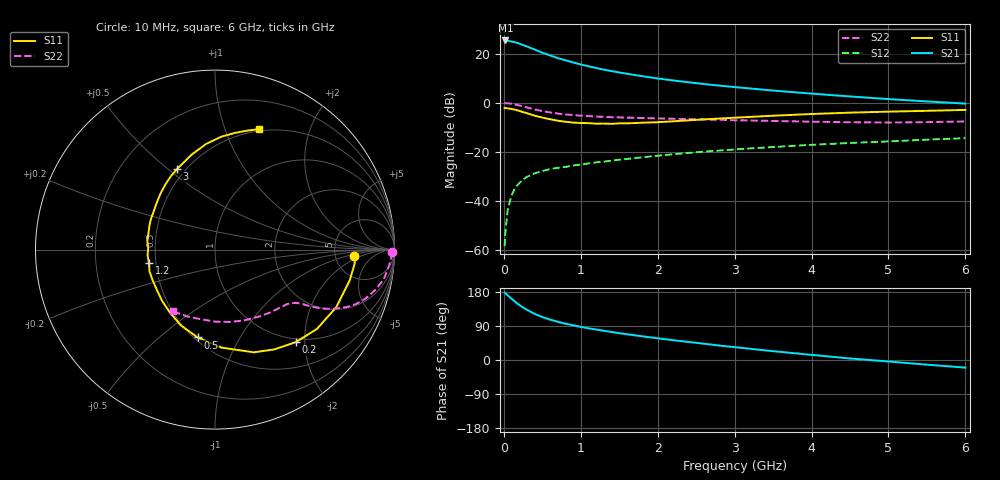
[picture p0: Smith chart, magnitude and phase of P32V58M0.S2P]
! SIEMENS Small Signal Semiconductors
! BFP181
! Si NPN RF Bipolar Junction Transistor in SOT143
! VCE = 2.5 V  IC = 8 mA
! Common Emitter S-Parameters:  March  1996
# GHz  S  MA  R  50
!  f  S11  S21  S12  S22
! GHz  MAG  ANG  MAG  ANG  MAG  ANG  MAG  ANG
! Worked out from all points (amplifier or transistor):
!   36 points, 10 MHz to 6 GHz, reference 50 ohm
!   highest |S21| = 25.4 dB at 20 MHz (marker M1)
!   |S21| within 3 dB of that: start of sweep to 344 MHz
!   unconditionally stable (mu >= 1): 1.239 GHz to end of sweep
!   at 250 MHz: K = 0.30, MSG = 27.4 dB, |S12| = -31.2 dB
!   at 1.4 GHz: K = 1.06, MAG = 16.8 dB, |S12| = -23.6 dB
!   at 6 GHz: K = 1.02, MAG = 6.3 dB, |S12| = -14.4 dB
!   S11 on the Smith chart (normalised r, x): 10 MHz: 7.65, -1.46; 200 MHz: 0.94, -1.81; 500 MHz: 0.52, -0.68; 1.2 GHz: 0.46, -0.08; 3 GHz: 0.45, +0.54; 6 GHz: 0.48, +1.32
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0.01  0.776 -2.8  18.5 178.0  0.0012 85.0  0.984 -0.9
0.02  0.7826 -5.5  18.59 176.5  0.0023 88.2  0.9854 -2.0
0.05  0.77 -12.8  18.36 170.6  0.0066 84.3  0.9749 -5.1
0.1  0.7479 -25.4  17.64 161.8  0.013 76.0  0.9548 -10.0
0.15  0.7198 -37.9  17.02 153.0  0.0189 71.1  0.9194 -14.3
0.2  0.6842 -48.9  16.09 145.4  0.023 66.0  0.882 -18.0
0.25  0.6469 -59.3  14.96 138.4  0.0274 62.9  0.8423 -21.1
0.3  0.6119 -69.3  14.03 132.5  0.031 59.1  0.8019 -23.5
0.4  0.5473 -86.2  12.13 121.7  0.0365 54.2  0.7321 -26.9
0.5  0.4989 -101.2  10.46 113.4  0.0406 50.1  0.6783 -28.9
0.6  0.463 -114.3  9.245 106.7  0.0446 48.4  0.6366 -30.2
0.7  0.4313 -125.5  8.128 100.9  0.0473 47.4  0.6037 -31.1
0.9  0.3949 -144.7  6.638 91.7  0.0527 46.1  0.5606 -32.4
1.1  0.3847 -161.6  5.551 83.6  0.0581 46.1  0.5347 -33.8
1.2  0.3755 -168.5  5.11 80.4  0.0611 45.6  0.525 -34.6
1.6  0.3812 166.9  3.9 68.0  0.0718 45.5  0.4986 -38.2
2.2  0.4191 140.2  2.849 52.3  0.0894 43.9  0.4726 -46.0
3  0.4964 115.2  2.088 33.9  0.112 39.7  0.4416 -58.6
3.5  0.5449 103.8  1.773 23.3  0.1257 36.5  0.4263 -67.9
4.5  0.6291 87.0  1.345 4.1  0.1516 29.1  0.4014 -89.6
5.5  0.6858 75.0  1.065 -12.3  0.1776 22.4  0.4033 -112.5
6  0.7152 69.8  0.962 -20.1  0.19 18.4  0.4161 -124.2
